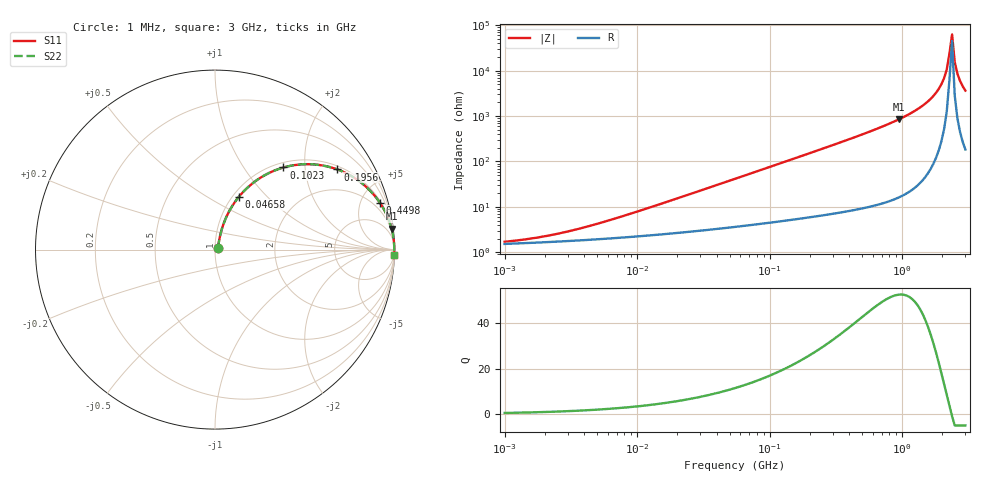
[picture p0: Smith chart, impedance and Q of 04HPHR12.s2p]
# MHz S MA R 50
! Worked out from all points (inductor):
!   174 points, 1 MHz to 3 GHz, reference 50 ohm
!   read as one part in series: L = 120 nH near 8.803 MHz
!   highest Q = 52.5 at 943.3 MHz (marker M1), where L = 143 nH
!   self-resonance near 2.273 GHz
!   S11 on the Smith chart (normalised r, x): 1 MHz: 1.03, +0.02; 46.58 MHz: 1.07, +0.70; 102.3 MHz: 1.09, +1.55; 195.6 MHz: 1.12, +2.97; 449.8 MHz: 1.17, +7.04; 3 GHz: 5, -73
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1  0.01676 25.9  0.9849 -0.4  0.9849 -0.4  0.01676 25.9
2.00209  0.02208 41.4  0.9836 -0.9  0.9836 -0.9  0.02208 41.4
3.8271  0.03358 55.9  0.9816 -1.6  0.9816 -1.6  0.03358 55.9
14.6467  0.1098 71.4  0.9705 -6.2  0.9705 -6.2  0.1098 71.4
46.5816  0.3232 65.7  0.9155 -18.8  0.9155 -18.8  0.3232 65.7
56.0545  0.3792 62.9  0.8933 -22.2  0.8933 -22.2  0.3792 62.9
102.305  0.5956 50.2  0.7693 -36.5  0.7693 -36.5  0.5956 50.2
195.561  0.8149 33.2  0.5485 -54.5  0.5485 -54.5  0.8149 33.2
214.526  0.8389 30.9  0.514 -57.0  0.514 -57.0  0.8389 30.9
449.846  0.9558 15.7  0.2715 -72.8  0.2715 -72.8  0.9558 15.7
821.013  0.9874 8.1  0.1401 -80.8  0.1401 -80.8  0.9874 8.1
943.294  0.9909 6.7  0.117 -82.2  0.117 -82.2  0.9909 6.7
1430.66  0.997 3.3  0.05837 -85.3  0.05837 -85.3  0.997 3.3
1888.56  0.9986 1.4  0.02512 -86.0  0.02512 -86.0  0.9986 1.4
2071.71  0.9988 0.8  0.01458 -84.8  0.01458 -84.8  0.9988 0.8
2169.84  0.9989 0.5  0.009371 -82.7  0.009371 -82.7  0.9989 0.5
2272.62  0.9989 0.2  0.004245 -74.5  0.004245 -74.5  0.9989 0.2
2380.27  0.9989 -0.1  0.001588 44.1  0.001588 44.1  0.9989 -0.1
2493.02  0.9988 -0.4  0.006418 79.2  0.006418 79.2  0.9988 -0.4
2611.11  0.9987 -0.7  0.01159 83.4  0.01159 83.4  0.9987 -0.7
2734.79  0.9986 -1.0  0.01681 84.8  0.01681 84.8  0.9986 -1.0
3000  0.9982 -1.6  0.02739 85.5  0.02739 85.5  0.9982 -1.6
